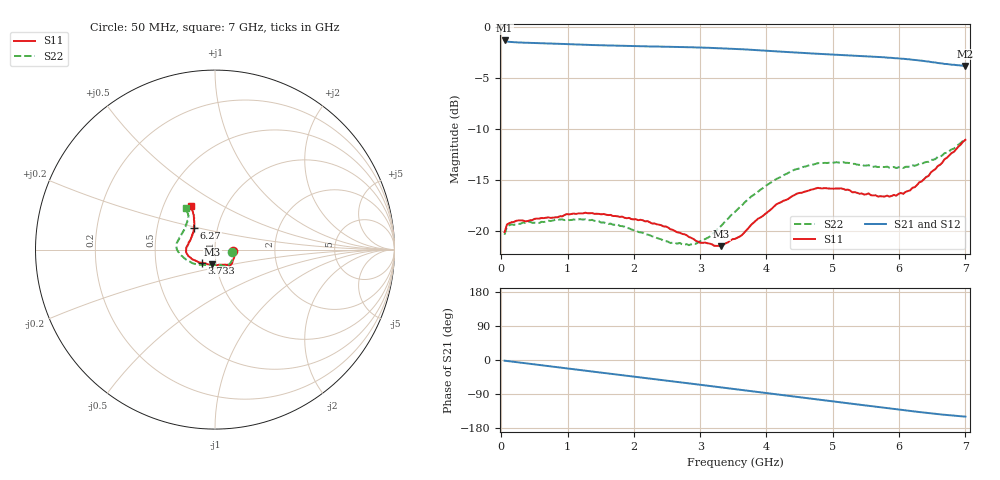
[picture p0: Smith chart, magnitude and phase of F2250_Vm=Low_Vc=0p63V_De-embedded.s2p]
! Integrated Device Technology
! Corporate Headquarters
! 6024 Silver Creek Valley Road
! San Jose, CA 95138  USA
! Phone:  1-408-284-8200
! Toll Free:  1-800-223-1366
! Webpage:  http://www.idt.com/
! Timing and RF Division
! 515 Groton Road, Suite 102
! Westford, MA 01886-6024
! Device:  F2250
! Description: Voltage Variable RF Attenuator
! Frequency:  50.0 -  6000.00 MHz
! Package:  3x3 mm Thin QFN Plastic Package: 16 pin
! Ports:  2 RF, 3 DC
!  Pin  1  = GND
!  Pin  2  = NC
!  Pin  3  = RF1  = Port 1
!  Pin  4  = NC
!  Pin  5  = GND
!  Pin  6  = GND
!  Pin  7  = GND
!  Pin  8  = GND
!  Pin  9  = NC
!  Pin 10  = RF2  = Port 2
!  Pin 11  = NC
!  Pin 12  = GND
!  Pin 13  = GND
!  Pin 14  = VCNTRL
!  Pin 15  = VDD
!  Pin 16  = VMODE
! Vcntrl:  0.630 Volts
! Vmode:  +0.000 Volts
! Vdd:  +3.30  Volts
! Current:  1.141 mA
! Data:  The device was measured on a the F2250 evaluation board which has
!  individual transmission lines to the RF pins.  Data was collected
!  using a calibrated network analyzer.  The evaluation board was
!  de-embedded using a TRL calibration technique.
!  The reference plane is the edge of the package pin.
! Misc:  SN 10
!  Action Tracker AT0258
! Date Measured:  2014-11-26
! Date:  2015-10-15  MJV
! Note:
!  Integrated Device Technology supplies this data as a sample of measured
!  data at the package pin for this product.  Your particular data for this
!  product may vary.
!  Data was taken at 25 degrees C.
!  Integrated Device Technology reserves the right to change this data at anytime.
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# GHz S dB R 50
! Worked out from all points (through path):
!   201 points, 50 MHz to 7 GHz, reference 50 ohm
!   highest |S21| = -1.36 dB at 50 MHz (marker M1); lowest = -3.9 dB at 7 GHz (marker M2)
!   group delay of S21, straight-line fit = 60 ps
!   lowest |S11| = -21.5 dB at 3.317 GHz (marker M3), VSWR 1.18, Z = 47.9 - j7.97 ohm
!   |S11| at or under -10 dB: start of sweep to end of sweep
!   |S22| runs from -21.4 to -11.0 dB; largest |S21 - S12| = 0.00057
!   S11 on the Smith chart (normalised r, x): 50 MHz: 1.22, -0.02; 3.733 GHz: 0.86, -0.13; 6.27 GHz: 0.77, +0.19; 7 GHz: 0.68, +0.36
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0.05  -20.15 -5.4  -1.36 -1.8  -1.36 -1.8  -20.40 -6.7
0.08475  -19.40 -5.7  -1.46 -2.5  -1.46 -2.5  -19.61 -6.5
0.15425  -19.17 -7.6  -1.52 -4.0  -1.52 -4.0  -19.39 -8.4
0.71025  -18.69 -27.3  -1.66 -16.2  -1.65 -16.2  -19.02 -31.9
1.2315  -18.30 -42.0  -1.78 -27.5  -1.78 -27.5  -18.91 -51.1
1.75275  -18.59 -48.8  -1.88 -38.5  -1.87 -38.5  -19.38 -61.6
2.37825  -19.41 -52.2  -1.96 -51.8  -1.96 -51.8  -20.79 -71.8
2.552  -19.86 -55.2  -1.98 -55.6  -1.98 -55.6  -21.21 -77.8
2.93425  -20.99 -69.5  -2.05 -64.0  -2.04 -64.0  -21.29 -98.7
3.14275  -21.27 -84.4  -2.09 -68.6  -2.08 -68.6  -20.59 -114.3
3.3165  -21.52 -100.1  -2.13 -72.5  -2.13 -72.5  -19.53 -125.5
3.525  -20.80 -118.1  -2.19 -77.1  -2.19 -77.1  -18.15 -137.6
3.7335  -19.71 -134.7  -2.26 -81.8  -2.26 -81.8  -16.87 -147.5
4.1505  -17.41 -155.3  -2.43 -91.0  -2.43 -91.0  -14.93 -165.1
4.46325  -16.36 -165.9  -2.55 -97.8  -2.55 -97.8  -13.95 -174.2
4.7065  -15.94 -172.8  -2.64 -103.0  -2.64 -103.0  -13.52 -179.8
5.15825  -15.91 176.0  -2.80 -112.7  -2.81 -112.7  -13.29 170.2
5.85325  -16.66 152.0  -3.05 -127.6  -3.05 -127.6  -13.83 154.1
6.06175  -16.39 143.4  -3.15 -132.1  -3.16 -132.1  -13.86 148.0
6.27025  -15.53 134.4  -3.29 -136.6  -3.30 -136.6  -13.57 141.4
6.61775  -13.55 123.3  -3.59 -143.3  -3.60 -143.3  -12.75 129.7
7  -11.10 119.1  -3.86 -149.5  -3.86 -149.5  -11.03 125.2
